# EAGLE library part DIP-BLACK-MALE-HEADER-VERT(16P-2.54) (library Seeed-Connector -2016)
320020034
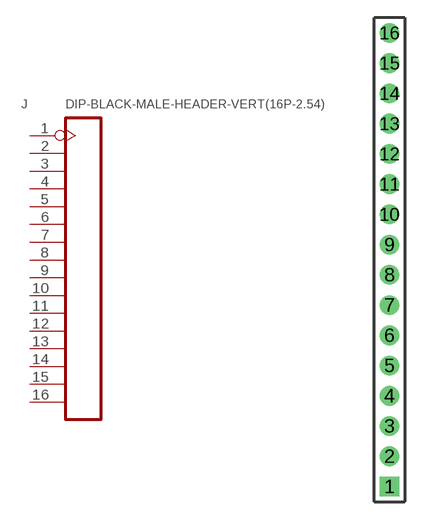
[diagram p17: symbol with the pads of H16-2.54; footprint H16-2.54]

Designator prefix J

## DIP-BLACK-MALE-HEADER-VERT(16P-2.54) (MPN: P125-1116A0BS116AX; VALUE: 16p-2.54)  [H16-2.54]
1  1  pas
2  2  pas
3  3  pas
4  4  pas
5  5  pas
6  6  pas
7  7  pas
8  8  pas
9  9  pas
10  10  pas
11  11  pas
12  12  pas
13  13  pas
14  14  pas
15  15  pas
16  16  pas

## Footprint H16-2.54 (pad centres in mm)
drill 0.889 pad 1.651 square: 1 0,-19.05
drill 0.889 pad 1.651: 2 0,-16.51; 3 0,-13.97; 4 0,-11.43; 5 0,-8.89; 6 0,-6.35; 7 0,-3.81; 8 0,-1.27; 9 0,1.27; 10 0,3.81; 11 0,6.35; 12 0,8.89; 13 0,11.43; 14 0,13.97; 15 0,16.51; 16 0,19.05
